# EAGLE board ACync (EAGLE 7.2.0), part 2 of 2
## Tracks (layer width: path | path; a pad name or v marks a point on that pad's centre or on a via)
16VAC
  Top 0.5: R46.1 13.88,51.88 13.88,55 D1.K+ 13.88,55.12 13.88,57.75 | 13.88,57.75 13.88,61 D2.A- | F1.2A 7.88,62.75 7.88,57.75 F1.2B 8.12,57.75 13.88,57.75
!ADC_CS  (via drill 0.51)
  Top 0.18: v267.88,41.88 267.88,40.88 267.38,40.38 v244.5,40.38 243,40.38 IC3.19 | v278.88,43.88 279.12,43.88 281,42 281,40.62 281.38,40.25 282.88,40.25 IC4.19 | v143.75,64 143.5,63.75 142.38,63.75 IC20.67 | v227.93,44.12 v195.64,44.12
  Bottom 0.18: v267.88,41.88 276.88,41.88 v278.88,43.88 | v195.64,44.12 163.38,44.12 156.64,50.86 156.64,59.64 155.64,60.64 147.36,60.64 144,64 v143.75,64 | v244.5,40.38 244.5,40.88 244.08,41.3 244.08,44.64 243,45.72 240.12,45.72 238.53,44.12 v227.93,44.12
!DAC_CS  (via drill 0.51)
  Top 0.18: v157.88,62.25 142.38,62.25 IC20.64 | v169.62,59.75 170.75,60.88 170.75,61.5 IC12.23
  Bottom 0.18: v169.62,59.75 160.38,59.75 v157.88,62.25
!DAC_LD  (via drill 0.51)
  Top 0.18: v155.62,65.5 152.88,62.75 142.38,62.75 IC20.65 | v165.25,65.5 169.5,69.75 169.5,70.38 IC12.7
  Bottom 0.18: v155.62,65.5 155.9,65.5 156.24,65.16 164.91,65.16 v165.25,65.5
!POT_STRT  (via drill 0.51)
  Top 0.18: v109.38,52.62 115,58.25 120.5,58.25 IC20.125 | v49,20.38 47.5,20.38 47.25,20.12 IC15.7
  Bottom 0.18: v109.38,52.62 101.2,52.62 101.2,52.6 97.2,48.6 97.2,41.76 95.76,40.32 92.07,40.32 71.12,19.38 50,19.38 v49,20.38
+1.2V  (via drill 0.51)  (1 unrouted)
  Top 0.25: v122.04,66.24 122.02,66.26 IC20.109 120.5,66.32 | IC20.102 126.11,66.85 v126.36,66.6 | IC20.116 121.44,62.76 v122.04,63.38 | IC20.124 121.24,58.76 121.68,58.59 v122.04,58.32 | IC20.138 121.42,51.76 v122.22,52.56 | IC20.5 125.11,47.69 v125.28,47.88 | IC20.1 123.11,47.51 v123.12,47.88 | IC20.29 137.11,47.83 v137.16,47.88 | IC20.45 140.96,52.76 v140.76,52.56 | IC20.78 138.11,67.09 v138.6,66.6 | IC20.84 135.11,66.71 v135,66.6 | C97.2 140.61,68.62 IC20.73 140.95,68.21 v141.12,68.04 | IC20.38 IC20.37 143.82,48.76 C86.2 | IC20.34 139.61,47.59 v139.32,47.88 | IC20.70 140.86,65.26 v140.76,65.16
  Top 0.4: 120.5,66.8 120.5,66.32
  Top 0.5: IC20.37 142.2,48.82 v142.2,48.96 | C50.2 101.12,62 101.12,65 C47.2 | C47.2 IC16.2 | C47.2 101.25,65.12 102.75,66.62 102.78,66.6 104.4,66.6 105.2,67.4 119.9,67.4 120.5,66.8
  Bottom 0.25: v122.04,66.24 C91.2 | v126.36,66.6 C90.2 | v122.04,63.38 C92.2 | v122.04,58.32 C94.2 | v122.22,52.56 C93.2 | v125.28,47.88 C83.2 | v123.12,47.88 C95.2 | v137.16,47.88 C85.2 | v140.76,52.56 C87.2 | v138.6,66.6 C89.2 | v135,66.6 C98.2 | v139.32,47.88 C96.2 | C88.2 140.72,65.2 v140.76,65.16
  Bottom 0.5: v122.04,58.32 120.96,59.4 120.96,63 121.32,63.36 122.02,63.36 v122.04,63.38 v122.04,66.24 122.04,66.96 122.76,67.68 125.62,67.68 126.36,66.94 v126.36,66.6 126.36,66.96 127.08,67.68 134.75,67.68 135.11,67.32 | C94.2 120.96,57.02 120.96,53.28 121.68,52.56 | 121.68,52.56 v122.22,52.56 | 121.68,52.56 120.96,51.84 120.96,48.96 122.04,47.88 v123.12,47.88 v125.28,47.88 126.36,46.8 136.75,46.8 137.11,47.16 137.11,47.83 v137.16,47.88 v139.32,47.88 141.12,47.88 v142.2,48.96 142.2,51.48 141.48,52.2 141.12,52.2 v140.76,52.56 | 135.11,67.32 135.47,67.68 137.86,67.68 138.6,66.94 v138.6,66.6 140.02,66.6 | 135.11,67.32 135.11,66.71 v135,66.6 | 140.02,66.6 140.76,65.86 v140.76,65.16 | 140.02,66.6 141.12,67.7 v141.12,68.04
+2.5V  (via drill 0.51, 0.71)  (1 unrouted)
  Top 0.25: 128.61,66.87 v128.88,66.6 | IC20.107 123.61,69.53 C78.2 | IC20.75 139.61,69.19 139.32,69.48 139.32,69.7 C81.2 | IC20.35 140.11,45.29 140.32,45.08 140.4,45 140.9,45 C80.2 | IC20.3 124.11,45.23 C84.2
  Top 0.5: R42.2A 135.62,33.25 136.38,33.25 R42.3A 136.38,33 136.38,32.62 136.75,32.25 137.62,32.25 138.88,33.5 138.88,33.75 140,34.88 C65.2 139.5,34.62 136.62,37.5 J15.4 136.62,37.75 137.75,38.88 137.75,41 138,41.25 | 138,41.25 140.25,43.5 140.25,45 140.32,45.08 | IC11.2 C39.2 101.12,54 101.12,51 C49.2 101,50.88 v101,50.45 | v123.5,70.62 123.5,69.62 C78.2 | v139.12,71 139.12,69.88 C81.2 | v124.38,43.88 124.38,45 C84.2 | v140,64.12 130.38,64.12 129,65.5 129,66.5 v128.88,66.6 | v135.12,44.12 138,41.25
  Bottom 0.25: v128.88,66.6 C82.2
  Bottom 0.5: v123.5,70.62 123.75,70.62 124.12,70.25 | 124.12,70.25 125.75,68.62 138,68.62 139.12,69.75 | v139.12,71 139.12,69.75 | v124.38,43.88 124.38,44.5 123,45.88 | 123,45.88 120.25,48.62 120.25,49.38 | 120.25,49.38 120.25,66.38 124.12,70.25 | v140,64.12 141,64.12 142.12,65.25 142.12,68.38 140.88,69.62 139.25,69.62 139.12,69.75 | v135.12,44.12 133.25,46 123.12,46 123,45.88 | 120.25,49.38 102.08,49.38 v101,50.45
+3.3V  (via drill 0.51, 0.71)
  Top 0.25: IC20.130 122,55.76 v122.04,55.8 | IC20.139 122,51.26 v122.04,51.3 | IC20.17 131.11,47.81 v131.04,47.88 | IC20.26 135.61,47.63 v135.36,47.88 | IC20.40 141.07,50.26 v140.76,49.95 | IC20.47 140.79,53.76 v140.76,53.73 | IC20.62 140.82,61.26 v140.76,61.2 | IC20.93 130.61,66.67 v130.68,66.6 | IC20.117 122.02,62.26 v122.04,62.28 | IC20.56 141.06,58.26 v140.76,57.96 | IC20.81 136.61,66.79 v136.8,66.6 | IC20.122 121.86,59.76 v122.04,59.94 | R61.1 112.81,49.55 113.04,49.32 113.04,48.44 IC18.7
  Top 0.5: C58.1 110.27,48.22 111.12,48.22 | 111.12,48.22 IC18.8 112.12,48.25 113.25,48.25 IC18.7 113.38,48 113.38,46.25 114,45.62 | IC4.18 280.37,39.67 280.08,39.96 280.08,42.12 279.27,42.92 IC4.2 275.02,42.92 C32.1 274.75,43.12 268.56,49.32 237.38,49.32 | C30.1 235.03,42.92 IC3.2 238.38,42.92 | 238.38,42.92 239.68,42.92 240.12,42.48 240.12,40.32 | 240.12,40.32 240.76,39.67 IC3.18 | C48.2 233,67 233,64.12 C38.2 IC10.2 235.62,63.88 236.62,62.88 236.75,62.88 237.38,62.25 237.38,49.32 | 238.38,42.92 238.38,44.62 237.38,45.62 237.38,49.32 | R17.CW 41.38,5.5 39.12,7.75 39.12,18 40.88,19.75 C41.1 41.11,20.06 IC15.2 43.38,20.12 43.88,20.12 44.74,20.98 44.74,22.42 49.82,27.5 56.74,27.5 57.6,26.64 57.6,24.48 58.32,23.76 84.24,23.76 86.4,25.92 97.42,25.92 102.75,31.25 104,31.25 111.88,39.12 | 114,45.62 114.5,45.12 114.5,44.25 IC18.3 | R55.3B 120.62,33.25 121.38,33.25 R55.2B | R55.2B 121.62,33.25 122.12,33.25 R55.1B 122.38,33.12 124,33.12 C59.2 124.12,33.25 126,33.25 | J15.6 134,37.62 133,36.62 C66.2 132.88,34.75 131.38,33.25 131.25,33.25 | 131.25,33.25 126,33.25 | 126,33.25 v126,34.25 | 111.12,48.22 111.12,39.88 111.88,39.12 | 111.88,39.12 118.75,32.25 120.25,32.25 121.12,33.12 R55.2B | 131.25,33.25 131.25,33.12 133.24,31.14 139.76,31.14 144.88,36.25 144.88,38.25 IC19.4 IC19.1 149.16,38.52 150.12,38.52 151,39.4 C67.1 153.45,40.05 156.35,42.95 C60.1 161.29,42.95 IC21.24 161.64,42.35 161.64,40.68 164.42,37.9 195.4,37.9 197.75,40.25 v212.88,40.25 | v122.12,49.62 122.12,48.75 120.75,47.38 120.75,46.62 119.88,45.75 114.12,45.75 114,45.62 | v239.38,40.25 239.88,40.25 240.12,40.32
  Bottom 0.25: v122.04,59.94 C68.2 | v122.04,55.8 C69.2 | v122.04,51.3 C70.2 | v131.04,47.88 C71.2 | v135.36,47.88 C72.2 | v140.76,49.95 C73.2 | v140.76,53.73 C74.2 | v140.76,61.2 C76.2 | v130.68,66.6 C79.2 | C63.2 v122.04,62.28 | C75.2 v140.76,57.96 | C77.2 v136.8,66.6
  Bottom 0.5: v122.04,59.94 122.04,60.84 | 122.04,60.84 v122.04,62.28 | 122.04,60.84 123.84,60.84 124.56,60.12 124.56,58.32 v122.04,55.8 124.56,53.28 124.56,51.12 | 122.4,50.4 123.84,50.4 124.56,51.12 | 124.56,51.12 126,51.12 129.24,47.88 v131.04,47.88 134.28,47.88 | v135.36,47.88 134.28,47.88 | 134.28,47.88 134.28,50.04 135.36,51.12 137.88,51.12 138.24,51.48 | v140.76,49.95 140.76,50.76 140.4,51.12 138.6,51.12 138.24,51.48 | 138.24,51.48 138.24,54 138.96,54.72 140.4,54.72 | 140.4,54.72 140.76,54.36 v140.76,53.73 | 140.4,54.72 140.76,55.08 v140.76,57.96 140.76,60.12 | v140.76,61.2 140.76,60.12 | C77.2 136.84,66.42 137.34,66.42 137.79,65.97 137.79,64.53 137.34,64.08 137.16,64.08 | 137.16,64.08 132.48,64.08 131.76,64.8 131.76,66.24 131.4,66.6 v130.68,66.6 | 122.4,50.4 122.04,50.76 v122.04,51.3 | v126,34.25 122.62,37.62 J16.4 | v122.12,49.62 122.25,49.75 122.25,50.25 122.4,50.4 | v212.88,40.25 v239.38,40.25 | 140.76,60.12 137.52,60.12 137.52,63.72 137.16,64.08
+5V  (via drill 0.71)
  Top 0.4: IC4.3 278.12,42.27 278.28,42.12 | IC3.3 238.16,42.27 238.32,42.12
  Top 0.5: C61.1 100.76,32.05 IC22.24 | IC24.8 189.95,46.19 C64.2 189.36,47.59 189.36,53.38 | C23.2 C33.1 274.98,39.02 IC4.8 278.06,39.02 278.28,39.24 278.28,40.12 | 278.28,42.12 278.28,40.12 | C31.1 234.97,39.02 IC3.8 238.1,39.02 238.32,39.24 238.32,42.12 | 28.05,28.88 28.05,28.29 IC23.8 | R39.1 21.62,33 23.3,31.32 26.64,31.32 26.95,31.01 C62.2 28.05,28.9 28.05,28.88 | 28.05,28.88 30.5,28.88 31.38,29.75 44.38,29.75 45,29.12 45,28.88 IC17.5 45,28.62 46.5,28.62 47,28.12 C100.2 47.12,28.25 57.07,28.25 58.32,27 58.32,24.84 58.68,24.48 83.88,24.48 86.04,26.64 96.84,26.64 100.44,30.24 100.44,31.94 100.5,32 IC22.24 | C29.2 99,57 IC11.3 96.4,58.68 95.4,58.68 | IC22.24 100.25,32.75 100.25,34.75 96.12,38.88 84.75,38.88 83.5,40.12 83.5,52.55 89.63,58.68 95.4,58.68 | C55.2 198,61 198,63 C40.2 | C55.2 198.12,61.5 201,61.5 IC5.3 201.12,61.25 206.38,56 235.12,56 | 189.36,53.38 178.88,53.38 175.38,56.88 173.25,56.88 172.25,57.88 C27.1 172.1,58.05 IC12.24 172.1,65.14 170.84,66.41 IC12.6 170.75,70.62 170.75,71.25 v169.62,72.38 | C19.2 235,37 235,38.88 C31.1 | C28.2 235,61 IC10.3 235.12,60.88 235.38,60.62 v235.38,58 235.12,57.75 235.12,56 | C31.1 234.88,39.25 234.88,41.38 234.12,42.12 234.12,44.75 235.12,45.75 235.12,56 | v278.38,40.12 278.28,40.12 | v122.75,77 110.12,77 101.25,68.12 C46.2 99,68 IC16.3 95.98,67.54 95.4,66.96 95.4,58.68 | C55.2 197.95,56.83 194.5,53.38 189.36,53.38
  Bottom 0.5: v122.75,77 123.25,77 124.75,78.5 163.5,78.5 v169.62,72.38 | v235.38,58 242.38,58 261.38,39 276,39 277.12,40.12 v278.38,40.12
+10V
  Top 0.18: IC13.1 181,71 R1.1 181,71.12 179,71.12 C34.2 179,71 178.5,70.5 177.25,70.5 IC12.1
+15V  (via drill 0.71)  (2 unrouted)
  Top 0.5: IC1.8 232.05,28.29 C1.2 232.25,30.12 233.25,31.12 238.75,31.12 242.25,34.62 C18.2 | IC14.8 252.05,28.29 C42.2 252.25,30.12 252.56,30.44 | IC2.8 272.03,29.98 C3.2 | IC9.8 292.05,28.29 291.87,28.47 C44.2 291.87,31.05 290.52,32.4 284.76,32.4 284.4,32.76 281.88,32.76 281.77,32.87 | IC4.15 282.17,37.73 281.88,37.44 281.88,35.17 C22.2 282,34.95 282,33.1 281.77,32.87 | IC3.15 242.21,37.73 241.92,37.44 | 241.92,37.44 241.92,35.13 C18.2 | C18.2 242.25,34.88 245.12,32 251,32 252.56,30.44 | C3.2 272.25,30.12 273.25,31.12 274.56,31.12 275.6,30.08 278.98,30.08 281.77,32.87 | 252.56,30.44 254.88,32.75 269.25,32.75 271.88,30.12 C3.2 | C56.2 74,55 72,55 C9.2 72.62,55.12 72.62,58 IC6.3 72.75,58.12 v83.28,58.12 | IC12.25 173.38,60.75 174,60.12 C35.2 174.12,58.12 183.38,58.12 183.5,58 185.38,58 195.62,68.25 | 197.88,66 195.62,68.25 | 195.62,68.25 189.88,74 v180,74 180.88,73.12 R1.2 181,72.88 | v239.62,37.5 241.75,37.5 241.92,37.44
  Bottom 0.5: v83.28,58.12 83.62,58.12 105.5,80 174,80 v180,74 180.12,73.88 180.12,67.5 210.12,37.5 v239.62,37.5
-10V
  Top 0.18: 181,61 IC8.2 | 181,61 179,61 | 181,61 R2.2 | 179,61 178.5,61.5 177.25,61.5 IC12.28 | 179,61 C36.2
-15V  (via drill 0.71)  (1 unrouted)
  Top 0.25: IC4.10 276.05,37.73 275.67,37.35 275.67,36.27 275.04,35.64 275.04,35.05 C25.1 | IC3.10 236.09,37.73 235.8,37.44 235.8,36 234.95,35.15 C21.1
  Top 0.5: IC1.4 227.95,24.44 C2.2 228.12,23.38 230.5,23.38 | 287.95,24.44 IC9.4 | 230.5,23.38 244.75,23.38 245.5,24.12 247.75,24.12 IC14.4 247.95,24.44 C43.2 248.12,23.5 253.25,23.5 253.8,24.05 253.8,24.48 254.16,24.84 266.4,24.84 266.78,24.46 IC2.4 267.95,24.44 C4.2 268.12,23.62 273.38,23.62 274,24.25 279.12,24.25 | 279.12,24.25 279.38,24.25 279.5,24.12 287.75,24.12 IC9.4 | 232.25,31.88 233.62,31.88 233.88,32.12 233.88,33.62 234.88,34.62 234.88,35 C21.1 | 232.25,31.88 230.5,30.12 230.5,23.38 | v278.38,37.12 277.75,37.75 277.12,37.75 IC4.10 | v279.12,24.5 279.12,24.25 | C57.1 66,49.12 68,49.12 C10.2 | C10.2 67.38,49 67.38,46 IC7.3 | R2.1 181,59.12 182.62,59.12 183.5,60 185.5,60 185.75,60.25 185.88,60.25 v186,60.12 186.35,60.48 186.84,60.48 190.08,63.72 190.08,64.08 187.16,67 176,67 173.38,69.62 IC12.4 173.25,70.62 173,70.88 173,74 C13.1 172.75,74.12 v171.38,75.5 | v74.25,49.88 69.12,49.88 68.25,49 C10.2 | v210.88,35.25 229.12,35.25 232.12,32.25 232.12,32 232.25,31.88 | C45.2 287.97,22.8 IC9.4
  Bottom 0.5: v74.25,49.88 76.73,49.88 106.11,79.25 167.62,79.25 v171.38,75.5 | v186,60.12 v210.88,35.25 | v278.38,37.12 280.44,35.06 280.44,26.28 279.12,24.96 v279.12,24.5
ADC1  (via drill 0.51)
  Top 0.18: v235.75,44.88 237,43.62 IC3.1 | v176.5,57.12 v193.88,57.12 | v149.62,64.75 142.38,64.75 IC20.69
  Bottom 0.18: v193.88,57.12 206.12,44.88 224.88,44.88 226.44,46.44 234.19,46.44 v235.75,44.88 | v176.5,57.12 168.88,64.75 v149.62,64.75
ADC2  (via drill 0.51)
  Top 0.18: v241.38,42.88 242.88,42.88 IC3.23 | v212.12,42.88 197.25,42.88 194.5,40.12 179.88,40.12 160.75,59.25 142.38,59.25 IC20.58
  Bottom 0.18: v241.38,42.88 234.75,42.88 234.36,42.48 212.52,42.48 v212.12,42.88
ADC3  (via drill 0.51)
  Top 0.18: v266,53.38 275.75,43.62 277,43.62 IC4.1 | v256.25,63.12 255.75,63.12 241.12,77.75 152.75,77.75 149,74 149,70.88 143.88,65.75 142.38,65.75 IC20.71
  Bottom 0.18: v256.25,63.12 v266,53.38
ADC4  (via drill 0.51)
  Top 0.18: IC4.23 282.88,43 281.75,43 266.62,58.12 259.12,58.12 239.88,77.38 152.97,77.38 149.4,73.8 149.4,70.15 v148.75,69.5 | IC20.72 143.66,66.26 146.52,69.12 146.52,69.45 v146.47,69.5
  Bottom 0.18: v146.47,69.5 v148.75,69.5
ADC_!START  (via drill 0.51)
  Top 0.18: 245.62,41.62 245.78,41.62 245.91,41.5 v264.15,41.5 | 245.62,41.62 IC3.21 | v277,44.62 279.5,44.62 282.5,41.62 IC4.21 | v152.5,63.5 152.25,63.25 142.38,63.25 IC20.66 | 245.62,41.62 v245.62,41.5 | v194,47.12 221.12,47.12 v222.12,46.12
  Bottom 0.18: v277,44.62 267.28,44.62 v264.15,41.5 | v222.12,46.12 222.12,46.45 224.28,48.6 243,48.6 245.52,46.08 245.52,41.6 v245.62,41.5 | v152.5,63.5 153,63 159.48,63 162,60.48 170.15,60.48 184.5,46.12 193,46.12 v194,47.12
ADC_SCLK  (via drill 0.51)
  Top 0.18: v267,41.12 266.62,40.75 245.25,40.75 244.88,41.12 244.12,41.12 244,41 243,41 IC3.20 242.88,41 242.38,41 v241.75,41.62 | v281.75,41 282.88,41 IC4.20 | v140.75,63.12 140.75,63.62 141.38,64.25 IC20.68 | v225.69,41.62 v198.5,41.62
  Bottom 0.18: 281.62,41.12 v281.75,41 279.91,42.84 278.64,42.84 277.2,41.4 268.92,41.4 268.64,41.12 v267,41.12 | v241.75,41.62 241.34,41.62 240.48,42.48 235.44,42.48 234.36,41.4 225.91,41.4 v225.69,41.62 | v198.5,41.62 197.06,41.62 195.12,43.56 163.31,43.56 156,50.88 156,59 155,60 147,60 144,63 140.88,63 v140.75,63.12
AGND  (via drill 0.51, 0.71)  (21 unrouted)
  Top 0.18: IC20.118 121.48,61.76 121.77,61.47 123.03,61.47 123.48,61.92 v123.48,62.28 | IC20.123 121.55,59.26 121.68,59.13 123.21,59.13 123.48,59.49 v123.48,59.94 | IC20.131 121.5,55.26 121.77,54.99 123.03,54.99 123.48,55.44 v123.48,55.8 | IC20.140 121.5,50.76 121.77,50.49 123.21,50.49 123.48,50.76 v123.48,51.3 | IC20.19 132.11,48.61 131.76,48.96 131.4,48.96 v131.04,49.32 | IC20.27 136.11,48.93 135.72,49.32 v135.36,49.32 | IC20.41 139.68,50.76 139.32,50.4 v139.32,50.04 140.61,48.75 IC20.36 140.93,46.41 C80.1 | IC20.48 141.31,54.26 141.03,54.54 139.86,54.54 139.32,54 v139.32,53.64 | IC20.57 139.76,58.76 139.32,58.32 v139.32,57.96 | IC20.63 141.28,61.76 141.03,62.01 139.77,62.01 139.32,61.56 v139.32,61.2 | IC20.79 137.61,65.61 137.16,65.16 v136.8,65.16 136.44,65.16 135.99,65.61 135.99,67.05 136.11,67.17 IC20.82 | IC20.95 129.61,65.87 130.32,65.16 v130.68,65.16 | v123.48,66.24 123.11,66.61 IC20.108 123.11,68.77 122.76,69.12 122.76,69.38 C78.1 | IC20.4 124.61,47.47 124.56,47.52 124.11,47.52 | 124.11,47.52 123.84,47.52 123.61,47.29 IC20.2 123.61,45.27 C84.1 | IC20.74 140.11,69.77 C81.1 140.4,69.62 C97.1 | v123.84,49.32 123.93,49.32 124.11,49.14 124.11,47.52 | 16COM.TP 6.12,34.2 | 2.52,34.2 16COM.TP | 16COM.TP 4.32,36 | 4.32,32.4 16COM.TP
  Bottom 0.18: C63.1 v123.48,62.28 123.26,62.5 C92.1 | v123.48,59.94 C68.1 C94.1 | C69.1 v123.48,55.8 | v123.48,51.3 C70.1 C93.1 | C71.1 v131.04,49.32 | C72.1 v135.36,49.32 135.58,49.1 C85.1 C96.1 | C73.1 v139.32,50.04 | C74.1 v139.32,53.64 139.54,53.42 C87.1 | C75.1 v139.32,57.96 | C76.1 v139.32,61.2 | C77.1 v136.8,65.16 | C79.1 v130.68,65.16 130.46,65.38 C82.1 C90.1 | C91.1 v123.48,66.24 | C95.1 123.62,49.1 v123.84,49.32 124.06,49.1 C83.1 | 139.32,48.96 v139.32,50.04 | 139.54,50.26 v139.32,50.04 | 137.02,65.38 v136.8,65.16 | 136.58,65.38 v136.8,65.16 | C89.1 138.78,65.2 138.92,65.2 | 138.92,65.2 C88.1 | 138.92,65.2 v138.96,65.16 | v135,65.16 C98.1
  other vias: 36,27 32.04,30.96 72.72,46.08 68.04,51.84 98.72,51.56 108.44,46.16 116,44 103.04,57.04 158.84,41.12 158.84,33.2 150.92,41.84 185.12,70.64 177.56,73.16 191.6,38.96 191.6,41.12 178.84,59.2 172,55.96 168.76,66.04 233,38.96 233,35 235.08,27.96 236.96,33.2 247.04,35 253.88,29.96 235.88,41.48 241.28,38.6 118.52,36.44 122.48,36.28 126.38,36.38 141.5,35.3 100.16,49.04 102.68,48.32 103.04,54.08 274.04,29.96 272.96,32.84 276.2,32.84 278.12,35.12 175.76,40.4 175.76,36.44 126.36,65.16 45.36,19.08 265.76,23.12 24.84,29.88 23.76,24.12
  pour Top (rank 2): 0,0 300,0 300,81 0,81
  pour Bottom (rank 2): 0,0 300,0 300,81 0,81
  pour Top (rank 2): 0,0 300,0 300,81 0,81
  pour Bottom (rank 2): 0,0 300,0 300,81 0,81
ASDO  (via drill 0.51)
  Top 0.18: IC20.6 125.62,46.38 125.62,43.88 123.38,41.62 116.25,41.62 115,40.38 J16.9 | v116.88,47 116.88,47.12 115.88,48.12 IC18.5
  Bottom 0.18: v116.88,47 116.88,42.25 115,40.38 J16.9
CONF_DONE  (via drill 0.51)
  Top 0.18: R55.2A 121.5,34.88 121.5,39.25 122.5,40.25 J16.3 | v123.62,74.38 124,74 128.62,74 131.12,71.5 131.12,68.25 IC20.92 | v115.12,59 114.62,59 107.62,52 v107.62,48.38 107.28,48.03 CNFDN.TP
  Bottom 0.18: v123.62,74.38 123.62,73.88 120.96,71.21 120.96,69.48 120.24,68.76 117.72,68.76 115.2,66.24 115.2,59.08 v115.12,59 | J16.3 122.5,40.38 122.5,42.5 118.44,46.56 118.44,48.24 118.08,48.6 107.85,48.6 v107.62,48.38
D0  (via drill 0.51)
  Top 0.18: v119.12,55.25 119.62,54.75 120.5,54.75 IC20.132 | v112.62,65.62 v111,64 | v164.62,74.62 168.25,71 168.25,70.5 IC12.8
  Bottom 0.18: v119.12,55.25 117.62,53.75 115.88,53.75 109.5,60.12 109.5,62.5 v111,64 | v164.62,74.62 162.62,76.62 148.25,76.62 147,77.88 124.88,77.88 v112.62,65.62
D1  (via drill 0.51)
  Top 0.18: v118.38,57.5 118.38,54.88 119,54.25 120.5,54.25 IC20.133 | v146.62,77.12 v146.56,75.62 | v165.75,72.25 167,71 167,70.5 IC12.9
  Bottom 0.18: v146.56,75.62 126,75.62 121.32,70.94 121.32,69.12 120.6,68.4 118.08,68.4 115.56,65.88 115.56,60.12 115.92,59.76 117.82,59.76 118.38,59.2 v118.38,57.5 | v146.62,77.12 147.12,77.12 148,76.25 161.75,76.25 v165.75,72.25
D2  (via drill 0.51)
  Top 0.18: v117.25,54.5 118,53.75 120.5,53.75 IC20.134 | v113.75,65.62 v110.25,62.12 | v161.25,75.5 165.75,71 165.75,70.5 IC12.10
  Bottom 0.18: v117.25,54.5 116.75,54.5 116.62,54.38 115.88,54.38 110.25,60 v110.25,62.12 | v161.25,75.5 148.12,75.5 147.25,76.38 123.89,76.38 113.75,66.23 v113.75,65.62
D3  (via drill 0.51)
  Top 0.18: v143.14,69.02 141.25,67.12 139.38,67.12 139.12,67.38 139.12,68.12 IC20.76 | v164.38,68.5 164.38,70.38 IC12.11
  Bottom 0.18: v143.14,69.02 143.88,69.75 143.88,69.88 144.25,70.25 157.38,70.25 161.38,66.25 162.12,66.25 v164.38,68.5
D4  (via drill 0.51)
  Top 0.18: v138.12,70.12 138.62,69.62 138.62,68.25 IC20.77 | v162.5,72.12 162.5,71.75 163.12,71.12 163.12,70.5 IC12.12
  Bottom 0.18: v138.12,70.12 138.12,71.12 138.25,71.25 138.25,71.38 139,72.12 v162.5,72.12
D5  (via drill 0.51)
  Top 0.18: v137.12,70.75 137.12,68.25 IC20.80 | v160,72.88 161.88,71 161.88,70.5 IC12.13
  Bottom 0.18: v137.12,70.75 137.88,71.5 137.88,71.62 138.75,72.5 159.62,72.5 v160,72.88
D6  (via drill 0.51)
  Top 0.18: v156.38,74.75 160.62,70.5 IC12.14 | IC20.83 135.62,68.25 135.62,71.38 135,72 133.94,72 v133.66,72.28
  Bottom 0.18: v156.38,74.75 153.5,74.75 152.75,74 135.38,74 v133.66,72.28
D7  (via drill 0.51)
  Top 0.18: v116.25,55.12 116.25,54.38 117.38,53.25 120.5,53.25 IC20.135 | v121.38,75.5 142.62,75.5 144.62,73.5 v144.62,69.5 | v147.5,66.62 156.34,66.62 160.68,62.3 IC12.15
  Bottom 0.18: v116.25,55.12 115.75,55.12 111.75,59.12 111.75,65.88 112.83,66.96 113.4,66.96 121.38,74.94 v121.38,75.5 | v147.5,66.62 v144.62,69.5
D8  (via drill 0.51)
  Top 0.18: v134.88,69.62 134.62,69.38 134.62,68.25 IC20.85 | v137.12,71.88 140,71.88 v140.5,71.38 | v152.62,71.38 161.88,62.12 161.88,61.62 IC12.16
  Bottom 0.18: v137.12,71.88 v134.88,69.62 | v152.62,71.38 v140.5,71.38
D9  (via drill 0.51)
  Top 0.18: v134.88,70.75 134.12,70 134.12,68.25 IC20.86 | v154.75,73.25 154.75,70.62 163.12,62.25 163.12,61.62 IC12.17
  Bottom 0.18: v134.88,70.75 137.38,73.25 v154.75,73.25
D10  (via drill 0.51)
  Top 0.18: v133.62,70.62 133.62,68.25 IC20.87 | v153.88,74 155.12,74 156,73.12 156,70.62 164.38,62.25 164.38,61.62 IC12.18
  Bottom 0.18: v133.62,70.62 136.25,73.25 136.75,73.25 137.12,73.62 153.5,73.62 v153.88,74
D11  (via drill 0.51)
  Top 0.18: v128.12,69.62 128.12,68.25 IC20.98 | v161.75,67 161.75,66.12 165.75,62.12 165.75,61.62 IC12.19 | v132.25,73.75 141.53,73.75 142.2,73.08 142.2,70.8 v142.38,70.62
  Bottom 0.18: v132.25,73.75 v128.12,69.62 | v142.38,70.62 158.12,70.62 v161.75,67
DAC_A0
  Top 0.18: IC20.59 142.38,59.75 168.38,59.75 169.5,60.88 169.5,61.5 IC12.22
DAC_A1
  Top 0.18: IC20.60 142.38,60.25 160.12,60.25 160.25,60.12 167.5,60.12 168.25,60.88 168.25,61.5 IC12.21
DATA0
  Top 0.18: IC20.13 129.12,46.38 129.12,44.5 126.12,41.5 126.12,39.5 125.88,39.25 124.38,39.25 123.5,40.12 123.5,40.75 123,41.25 118.38,41.25 117.5,40.38 J16.7 117.38,40.25 116.38,39.25 114.5,39.25 113.38,40.38 113.38,44.12 IC18.2
DCLK  (via drill 0.51)
  Top 0.18: IC20.12 128.62,46.38 128.62,44.62 125.12,41.12 125.12,40.38 J16.1 | v119.75,47 117.12,49.62 115.25,49.62 114.62,49 114.62,48.25 IC18.6
  Bottom 0.18: v119.75,47 119.75,46.5 125,41.25 125,40.38 J16.1
N$1
  Top 0.18: IC3.16 244.38,38.38 245,39 C20.2
N$2
  Top 0.18: IC3.9 237.5,38.38 239.62,36.25 239.62,33.62 239,33 C11.2
N$3  (via drill 0.51)
  Top 0.18: 238.31,36.31 238.88,35.75 238.88,35 C14.2 | 238.31,36.31 237.62,37 237.12,37 IC3.11 | v228,32 R5.2 | v238.25,36.25 238.31,36.31
  Bottom 0.18: v228,32 234,32 v238.25,36.25
N$4  (via drill 0.51)
  Top 0.18: 245,37 243,37 IC3.14 | v241.88,31.88 236,26 R6.2 | 245,37 v246,36 | 245,37 C15.2
  Bottom 0.18: v246,36 v241.88,31.88
N$5
  Top 0.18: IC3.13 243,36.38 244,36.38 245,35.38 245,35 R14.2
N$6
  Top 0.18: IC3.12 236.94,36.42 236.16,35.64 236.16,34.21 R7.2
N$7
  Top 0.18: IC3.22 246.28,42.27 BUSY2.TP
N$8
  Top 0.18: R5.1 228,28.38 IC1.1 228,28.25 228,27 IC1.2
N$9  (via drill 0.51)
  Top 0.18: C51.2 244.12,29 244.12,27 R20.2 244,27 v244,25.5 | R12.2 235,13 234,12 230.09,12 J1.LWR-CTR
  Bottom 0.18: v244,25.5 244,24.38 231.62,12 230,12 J1.LWR-CTR
N$10
  Top 0.18: R6.1 232.38,26 232.12,25.75 IC1.6 232.12,25.88 232.12,27 IC1.7
N$11
  Top 0.18: R3.2 230,21 228.5,21 226.75,22.75 226.75,23.75 226.5,24 226.5,24.88 227.25,25.62 227.88,25.62 IC1.3
N$12  (via drill 0.51)
  Top 0.18: v237.12,22.38 238.5,21 250,21 R4.2 | v235.12,24.38 232.12,24.38 IC1.5
  Bottom 0.18: v235.12,24.38 v237.12,22.38
N$13  (1 unrouted)
  Top 0.18: J2.UPR-CTR R4.1
N$14  (1 unrouted)
  Top 0.18: J1.UPR-CTR R3.1
N$15  (via drill 0.51)
  Top 0.18: 256,26 256,28 C52.2 | v257,26 256,26 | 256,26 R21.2 | R13.2 255,13 254,12 250.09,12 J2.LWR-CTR
  Bottom 0.18: v257,26 257,20.5 251.12,14.62 251.12,13.12 250,12 J2.LWR-CTR
N$16
  Top 0.18: R21.1 252.38,26 252.12,25.75 IC14.6
N$17
  Top 0.18: R23.1 292.38,26 292.12,25.75 IC9.6
N$18  (via drill 0.51)
  Top 0.18: v237.62,20.75 R12.1 | C51.1 245.88,29 v245,28.12 245.38,28.38 247.88,28.38 IC14.1
  Bottom 0.18: v245,28.12 243.12,28.12 241,26 241,24.12 v237.62,20.75
N$19  (via drill 0.51)
  Top 0.18: v255,23.25 R13.1 | v255,27.12 254.12,28 C52.1 254,28 253,27 IC14.7
  Bottom 0.18: v255,27.12 v255,23.25
N$20
  Top 0.18: IC9.2 R22.1
N$21
  Top 0.18: IC14.2 R20.1
N$22  (via drill 0.51)
  Top 0.18: C53.2 284.12,29 284.12,27 R22.2 284,27 v284,25.5 | R18.2 275,13 274,12 270.09,12 J3.LWR-CTR
  Bottom 0.18: v284,25.5 284,20.38 275.62,12 270,12 J3.LWR-CTR
N$23
  Top 0.18: C54.2 296,28 296,26 R23.2 295.88,26 295.88,20.14 295,19.27 R19.2 295,13.38 293.62,12 290,12 J4.LWR-CTR
N$24  (via drill 0.51)
  Top 0.18: v276.19,20.75 R18.1 | IC9.1 285.84,28.27 | 285.84,28.27 285.14,28.27 v285,28.12 | C53.1 285.95,28.38 285.84,28.27
  Bottom 0.18: v285,28.12 284.95,28.08 283.32,28.08 282.24,27 282.24,22.32 280.67,20.75 v276.19,20.75
N$25
  Top 0.18: R19.1 295,27.12 294.12,28 C54.1 293.05,27 IC9.7
N$26  (via drill 0.51)  (2 unrouted)
  Top 0.18: v249.75,24.5 252,24.5 IC14.5 | v176.88,68 176.88,69 176,69.88 176,70.38
  Bottom 0.18: v249.75,24.5 249.75,27.25 247,30 213,30 196.56,46.44 196.56,47.36 192.44,51.48 191.52,51.48 176.88,66.12 v176.88,68
N$27  (via drill 0.51)  (2 unrouted)
  Top 0.18: v236.62,24.75 244.38,24.75 245.25,25.62 247.88,25.62 IC14.3 | v175.88,68.62 174.75,69.75 174.75,70.38
  Bottom 0.18: v236.62,24.75 237,25.12 237,26 236.12,26.88 215.38,26.88 215.38,26.91 196.2,46.08 196.2,47.16 192.24,51.12 191.16,51.12 175.88,66.41 v175.88,68.62
N$28  (via drill 0.51)  (2 unrouted)
  Top 0.18: v278.12,27 280.38,24.75 284.38,24.75 285.25,25.62 287.88,25.62 IC9.3 | v187.08,63 176.88,63 176,62.12 176,61.62
  Bottom 0.18: v278.12,27 265.12,27 251,41.12 251,44 243,52 233,52 222,63 v187.08,63
N$29  (via drill 0.51)  (2 unrouted)
  Top 0.18: v290.83,24.32 291.38,24.5 292,24.5 IC9.5 | v185.84,64.95 177.46,64.95 174.75,62.25 174.75,61.62
  Bottom 0.18: v185.84,64.95 273.92,64.95 290.83,48.05 v290.83,24.32
N$30
  Top 0.18: IC4.16 284.75,38.38 285,38.62 C24.2
N$31
  Top 0.18: IC4.9 278.38,38.38 279.25,37.5 279.25,34.25 278,33 C12.2
N$32  (via drill 0.51)
  Top 0.18: IC4.11 276.48,37.08 276.12,36.72 276.12,35.15 C16.2 275.88,34.88 275.88,34.5 275.38,34 v271.88,34 | v268.88,31 268,31.88 R10.2
  Bottom 0.18: v271.88,34 v268.88,31
N$33  (via drill 0.51)
  Top 0.18: 285,37 283,37 IC4.14 | 285,37 v286,36 | R11.2 276,26 278,28 280,28 v283,31 | 285,37 C17.2
  Bottom 0.18: v286,36 283,33 v283,31
N$34
  Top 0.18: IC4.13 283,36.38 284,36.38 285,35.38 285,35 R16.2
N$35
  Top 0.18: IC4.12 277.07,32.27 276.48,31.68 275.76,31.68 275.04,32.4 275.04,32.91 R15.2
N$36
  Top 0.18: IC4.22 286.27,42.27 BUSY3.TP
N$37
  Top 0.18: R10.1 268,28.38 IC2.1 268,28.25 268,27 IC2.2
N$38
  Top 0.18: R11.1 272.38,26 272.12,25.75 IC2.6 272.12,25.88 272.12,27 IC2.7
N$39  (via drill 0.51)
  Top 0.18: v270,21.18 R8.2 | IC2.3 268,25.62 269.57,25.62 v269.64,25.56
  Bottom 0.18: v269.64,25.56 270,25.2 v270,21.18
N$40  (via drill 0.51)
  Top 0.18: v280,22.25 281.25,21 290,21 R9.2 | v277,25.25 276.62,25.25 276.25,24.88 272.5,24.88 272.12,24.5 IC2.5
  Bottom 0.18: v280,22.25 277.63,22.25 277.2,22.68 277.2,25.05 v277,25.25
N$41  (1 unrouted)
  Top 0.18: J4.UPR-CTR R9.1
N$42  (1 unrouted)
  Top 0.18: J3.UPR-CTR R8.1
N$43  (via drill 0.51)
  Top 0.18: v138.88,43.5 138.12,44.25 138.12,46.38 IC20.31 | IC21.23 163,42.5 163,43.48 160.09,46.4 154.77,46.4 v151.88,43.5
  Bottom 0.18: v151.88,43.5 v138.88,43.5
N$44
  Top 0.18: IC20.39 142.38,49.75 158.34,49.75 164.25,43.84 164.25,42.5 IC21.22
N$45
  Top 0.18: IC20.42 142.38,51.25 158.46,51.25 165.5,44.2 165.5,42.5 IC21.21
N$46
  Top 0.18: IC20.43 142.38,51.75 158.84,51.75 166.75,43.84 166.75,42.5 IC21.20
N$47
  Top 0.18: J6.LWR-CTR 14.07,11.91 15.12,12.96 15.12,19.13 R51.2
N$48
  Top 0.18: R51.1 15,34.38 16.38,35.75 57.75,35.75 58.32,35.18 58.32,33.48 63.67,28.12 80.12,28.12 87.12,35.12 98.12,35.12 99,34.25 99,32.62 IC22.23
N$49
  Top 0.18: J14.LWR-CTR 63.91,11.91 65,13 R29.2
N$50
  Top 0.18: J13.LWR-CTR 83.91,11.91 85,13 R28.2
N$51
  Top 0.18: J12.LWR-CTR 103.91,11.91 105,13 R27.2
N$52
  Top 0.18: J11.LWR-CTR 123.91,11.91 125,13 R26.2
N$53
  Top 0.18: J10.LWR-CTR 143.91,11.91 145,13 R25.2
N$54
  Top 0.18: J9.LWR-CTR 163.91,11.91 165,13 R41.2
N$55
  Top 0.18: J8.LWR-CTR 183.91,11.91 185,13 R53.2
N$56  (1 unrouted)
  Top 0.18: J14.UPR-CTR R44.1
N$57
  Top 0.18: R31.2 200,21 185.88,21 185.47,21.41 183.11,21.41 172,32.52 172,33.5 IC21.9
N$58
  Top 0.18: J7.LWR-CTR 203.91,11.91 205,13 R52.2
N$59  (via drill 0.51)
  Top 0.18: R52.1 201.25,20.75 200.5,20 197,20 186,9 157.88,9 v148.88,18 | IC22.22 97.75,30.75 v97,30
  Bottom 0.18: v97,30 96.84,29.84 96.84,25.56 99,23.4 106.92,23.4 110.32,20 146.88,20 v148.88,18
N$60  (via drill 0.51)
  Top 0.18: R53.1 182.88,20.75 171.25,32.38 171.25,34.88 171.12,35 149.25,35 142.75,28.5 128,28.5 125.88,30.62 v109.75,30.62 | v97.75,34.38 96.5,33.12 96.5,32.62 IC22.21
  Bottom 0.18: v109.75,30.62 101.5,30.62 v97.75,34.38
N$61  (via drill 0.51)
  Top 0.18: IC22.20 95.2,31.67 v96.12,30.75 | R41.1 164.75,21 v164.75,21.75
  Bottom 0.18: v96.12,30.75 97.38,30.75 97.92,30.2 97.92,25.56 99.36,24.12 107.28,24.12 110.65,20.75 163.75,20.75 v164.75,21.75
N$62  (via drill 0.51)
  Top 0.18: v140.75,16.5 R25.1 | IC22.19 94,32.5 94,31.25 v94.5,30.75
  Bottom 0.18: v140.75,16.5 140.33,16.92 104.5,16.92 104.14,17.28 104.14,21.14 103.68,21.6 102.96,21.6 102.6,21.24 94.32,21.24 93.6,21.96 93.6,29.85 v94.5,30.75
N$63  (via drill 0.51)
  Top 0.18: v117.62,28.12 R26.1 | v96,34.25 92.93,34.25 92.67,33.98 IC22.18
  Bottom 0.18: v96,34.25 101.81,28.44 117,28.44 117.31,28.12 v117.62,28.12
N$64  (via drill 0.51)
  Top 0.18: v103.38,20.75 R27.1 | IC22.17 91.39,31 91.8,30.6 93.22,30.6 v93.38,30.75
  Bottom 0.18: v103.38,20.75 94.09,20.75 93.24,21.6 93.24,30.61 v93.38,30.75
N$65  (via drill 0.51)
  Top 0.18: v87.75,23.5 R28.1 | IC22.16 90.12,31.45 88.2,29.52 87.86,29.52 v87.75,29.62
  Bottom 0.18: v87.75,29.62 v87.75,23.5
N$66  (via drill 0.51)
  Top 0.18: v77.62,20.75 R29.1 | IC22.15 88.86,31.25 88.2,30.6 87.78,30.6 v87.62,30.75
  Bottom 0.18: v87.62,30.75 v77.62,20.75
N$67  (1 unrouted)
  Top 0.18: J13.UPR-CTR R56.1
N$68  (via drill 0.51)
  Top 0.18: v127.12,72.38 127.12,68.25 IC20.100 | v126.25,74.75 124.38,74.75 124,75.12 122.12,75.12 121.52,74.52 120.96,74.52 119.88,75.6 116.64,75.6 115.42,74.38 v115.25,74.38 | v90.12,43.25 88.88,42 88.88,41.5 IC22.10
  Bottom 0.18: v127.12,72.38 127.12,73.88 v126.25,74.75 | v115.25,74.38 90.12,49.25 v90.12,43.25
N$69  (via drill 0.51)
  Top 0.18: v125.88,69.88 125.62,69.62 125.62,68.25 IC20.103 | v116.45,65.62 114.88,65.62 114.05,64.8 113.56,64.8 111,62.23 111,61.75 104.5,55.25 97.38,55.25 96.45,54.33 96.45,48.33 90.12,42 IC22.9
  Bottom 0.18: v125.88,69.88 125.5,69.88 123.88,71.5 123.12,71.5 121.68,70.06 121.68,68.76 120.96,68.04 118.44,68.04 116.45,66.05 v116.45,65.62
N$70  (via drill 0.51)
  Top 0.18: v115.25,71.62 117.62,74 118.38,74 119.75,72.62 124.27,72.62 125.12,71.77 125.12,68.25 IC20.104 | v92.62,43.25 91.5,42.12 91.5,41.5 IC22.8
  Bottom 0.18: v115.25,71.62 92.62,49 v92.62,43.25
N$71  (via drill 0.51)
  Top 0.18: v93.88,43.25 92.75,42.12 92.75,41.5 IC22.7 | IC20.105 124.62,68.25 124.62,69.88 124.75,70 124.75,71.52 124.27,72 119.16,72 118,73.16 v118,73.25
  Bottom 0.18: v118,73.25 115.27,70.52 114.77,70.52 93.88,49.62 v93.88,43.25
N$72  (via drill 0.51)
  Top 0.18: v119.88,69.62 121.75,71.5 123.88,71.5 124.38,71 124.38,70.25 124.12,70 124.12,68.25 IC20.106 | IC22.6 94,41.5 94,42 99.88,47.88 100.75,47.88 101.88,49 101.88,51.38 112.5,62 112.61,62 v112.86,62.25
  Bottom 0.18: v119.88,69.62 119.88,69.47 119.52,69.12 117.36,69.12 114.84,66.6 114.84,63 114.12,62.28 112.89,62.28 v112.86,62.25
N$73
  Top 0.18: IC20.110 118.68,65.76 104.76,51.84 104.76,46.8 104.04,46.08 98.64,46.08 95.4,42.84 95.4,41.61 IC22.5
N$74
  Top 0.18: IC20.111 120.5,65.25 119,65.25 105.12,51.37 105.12,46.44 104.4,45.72 99.47,45.72 96.5,42.75 96.5,41.5 IC22.4
N$75
  Top 0.18: IC20.44 142.38,52.25 159.24,52.25 168,43.48 168,42.5 IC21.19
N$76
  Top 0.18: IC20.112 120.5,64.75 119.12,64.75 105.48,51.1 105.48,46.08 104.76,45.36 99.73,45.36 97.75,43.38 97.75,41.5 IC22.3
N$77
  Top 0.18: IC20.46 142.38,53.25 159.12,53.25 169.38,43 169.38,42.5 IC21.18
N$78
  Top 0.18: IC20.113 120.5,64.25 119.25,64.25 105.84,50.84 105.84,45.72 105.12,45 100,45 99.12,44.12 99.12,41.5 IC22.2
N$79
  Top 0.18: IC20.54 142.38,57.25 145.07,57.25 147.5,54.82 159.18,54.82 170.62,43.38 170.62,42.5 IC21.17
N$80
  Top 0.18: IC20.55 142.38,57.75 145.29,57.75 147.86,55.18 159.82,55.18 171.88,43.12 171.88,42.5 IC21.16
N$81
  Top 0.18: R39.2 19.12,33 19.12,31.75 20.88,30 R40.2 | IC23.6 28,25.75 27.38,25.75 25.38,27.75 25.38,28.62 25,29 22,29 21,30 R40.2 | 20.88,30.12 R40.2
N$82
  Top 0.18: R40.1 19.12,30 19.12,28.75 20.88,27 R24.2 IC23.2
N$83  (via drill 0.51)
  Top 0.18: v115.62,26 109.62,20 64.62,20 63.75,20.88 60,20.88 R44.2 | v155.88,26 163,33.12 163,33.5 IC21.2
  Bottom 0.18: v155.88,26 v115.62,26
N$84
  Top 0.18: R56.2 80,21 84.12,21 87.5,24.38 88.22,24.38 90.47,22.12 109.88,22.12 117,29.25 118.62,29.25 124.12,23.75 155,23.75 164.25,33 164.25,33.5 IC21.3
N$85
  Top 0.18: R57.2 100,21 102.5,21 103.25,21.75 110.12,21.75 117.25,28.88 118.23,28.88 123.73,23.38 156,23.38 165.5,32.88 165.5,33.5 IC21.4
N$86
  Top 0.18: R58.2 120,20.88 123.75,20.88 124.5,20.12 125.75,20.12 128.25,22.62 156.5,22.62 166.75,32.88 166.75,33.5 IC21.5
N$87
  Top 0.18: R59.2 140,21 140.12,21 141.38,22.25 157.38,22.25 168,32.88 168,33.5 IC21.6
N$88
  Top 0.18: R60.2 160,21 161.38,21 169.38,29 169.38,33.5 IC21.7
N$89
  Top 0.18: R30.2 180,23 170.75,32.25 170.75,33.5 IC21.8
N$90
  Top 0.18: 28.12,23.75 28.12,24.38 IC23.5 | 28.12,23.75 28.12,21.5 29.5,20.12 30.5,20.12 31.25,20.88 33,20.88 R38.2 | 28.12,23.75 26.25,25.62 24,25.62 IC23.3
N$91
  Top 0.18: R38.1 33,19.12 35,19.12 R37.2 34.92,18.97 34.92,13.32 33.51,11.91 J5.LWR-CTR
N$92  (via drill 0.51)
  Top 0.18: v28.12,31.38 28.12,33 R35.2 | v31.25,28.25 31.25,27.62 31.88,27 R33.2 | v143.75,55.25 143.25,55.75 142.38,55.75 IC20.51 | v101.88,27.38 100.25,27.38 97.66,24.78 87.06,24.78 84.96,22.68 56.45,22.68 v53.62,25.5
  Bottom 0.18: v28.12,31.38 v31.25,28.25 34,25.5 v53.62,25.5 | v143.75,55.25 146,55.25 155.38,45.88 155.38,38 144.75,27.38 v101.88,27.38
N$93  (via drill 0.51)
  Top 0.18: v25.92,33 R34.2 | v33,28 34,27 R36.2 | v146.12,54 143.88,56.25 142.38,56.25 IC20.52 | v102.12,29.25 101.5,29.25 97.42,25.17 86.73,25.17 84.6,23.04 57.6,23.04 56.52,24.12 56.52,26.23 v56.5,26.25
  Bottom 0.18: v25.92,33 28,33 v33,28 34.85,26.15 37.45,26.15 37.55,26.25 v56.5,26.25 | v102.12,29.25 146,29.25 155,38.25 155,45.12 v146.12,54
N$94  (via drill 0.51)
  Top 0.18: v57.38,35 44,35 R49.1 | v119,44.12 122.38,47.5 122.38,48.25 123,48.88 123,49.62 126.88,53.5 138.12,53.5 139.88,55.25 IC20.50 | v94.33,37.22 79.97,37.22 v79.25,36.5
  Bottom 0.18: v57.38,35 77.75,35 v79.25,36.5 | v94.33,37.22 112.97,37.22 115,39.25 115.01,39.24 115.56,39.24 115.92,39.6 115.92,40.68 119,43.76 v119,44.12
N$95  (via drill 0.51)
  Top 0.18: v143.75,54.12 143.12,54.75 142.38,54.75 IC20.49 | R50.1 42,34.88 42.27,34.88 43.03,34.11 57.12,34.11 63.48,27.75 82.38,27.75 v84.38,29.75
  Bottom 0.18: v84.38,29.75 84.88,29.75 90.62,35.5 99.5,35.5 102.6,32.4 144.36,32.4 145.08,33.12 149.04,33.12 154.44,38.52 154.44,45 146.52,52.92 144.96,52.92 v143.75,54.12
N$96
  Top 0.18: 43.12,31.88 43.12,32.12 44,33 R49.2 | 43.12,31.88 43.12,31.38 IC17.3 | 43.12,31.88 42,33 R50.2
N$97  (1 unrouted)
  Top 0.18: J12.UPR-CTR R57.1
N$98  (1 unrouted)
  Top 0.18: J6.UPR-CTR R45.1
N$99  (via drill 0.51)
  Top 0.18: R54.1 30.5,20.75 34.75,25 39.38,25 43,28.62 IC17.4 43.12,28.75 v44,28.75 | IC17.1 45,31.25 45.33,31.25 v45.38,31.2
  Bottom 0.18: v44,28.75 44,29.83 v45.38,31.2
N$100  (via drill 0.51)
  Top 0.18: v24.08,33 R34.1 | v24.08,28.25 24,28.38 IC23.1
  Bottom 0.18: v24.08,33 23.4,32.32 23.4,29.16 24.08,28.48 v24.08,28.25
N$101
  Top 0.18: IC23.7 R33.1
N$102
  Top 0.18: 60HZ.TP 184.97,47.67 IC24.1 184.88,45.25 182,45.25 | 182,45.25 182,46 R43.1 | 182,45.25 182,44 R32.2
N$103
  Top 0.18: R48.2 191.25,43 189.75,41.5 189.12,41.5 IC24.5 189,41.5 186.88,41.5 185.75,42.62 185,42.62 IC24.3 184.88,42.75 181.75,42.75 180.5,44 R32.1
N$104  (via drill 0.51)
  Top 0.18: R43.2 180.12,46 180.12,48 R47.2 180,48 v177.75,50.25 | IC20.53 142.38,56.75 144.85,56.75 147.6,54 v158.88,54
  Bottom 0.18: v158.88,54 174,54 v177.75,50.25
N$105  (1 unrouted)
  Top 0.18: J11.UPR-CTR R58.1
N$106  (via drill 0.51)
  Top 0.18: 194,43 D3.3 | v148.5,77.5 147.12,78.88 23.8,78.88 16.2,71.28 16.2,51.12 15.05,49.97 R46.2 | 193.88,45 C99.2 | 194,43 194,45 C99.2 | 194,43 R48.1 | v191.16,48.88 192.32,47.71 192.32,46.72 193.95,45.09 C99.2
  Bottom 0.18: v148.5,77.5 163.25,77.5 167.76,72.99 167.76,72 190.88,48.88 v191.16,48.88
N$107  (via drill 0.51)
  Top 0.18: v137.38,45 134.75,45 134.12,45.62 134.12,46.38 IC20.23 | v143.25,44.25 144.25,44.25 144.88,43.62 IC19.3
  Bottom 0.18: v137.38,45 138,45 138.75,44.25 v143.25,44.25
N$108
  Top 0.5: 16VAC.TP 4.32,38.95 F1.1A 7.88,42.62 7.88,47.5 F1.1B
N$109
  Top 0.18: J5.UPR-CTR R54.2
N$110
  Top 0.18: IC15.8 49.33,21.33 BUSY1.TP
N$111
  Top 0.5: D1.A- 23.75,55 C8.NEG 32.12,46.62 41.21,46.62 45.8,42.03 70,42.03 | C6.2 IC7.2 70,42.03 | IC7.TAB 70,42.03
N$112
  Top 0.5: C5.2 68,57.5 67.5,58 IC6.1 67.25,58.12 52.12,58.12 C7.POS 46,64.25 23.62,64.25 20.38,61 D2.K+
N$113
  Top 0.18: IC15.1 43.12,21.25 43,21.12 39,21.12 C26.2 39,18.62 38.5,18.12 38.5,5.25 40.5,3.25 42.38,3.25 46.5,7.38 46.5,8 R17.W
N$114  (via drill 0.51)
  Top 0.18: v139.12,45 139.12,46.38 IC20.33 | IC21.15 173.12,42.5 173.12,43.12 160.71,55.54 148.68,55.54 148.44,55.78 v148.44,57.5
  Bottom 0.18: v139.12,45 139.38,45 143,48.62 143,51.76 141.58,53.18 141.58,57.24 141.94,57.6 148.34,57.6 v148.44,57.5
N$115  (1 unrouted)
  Top 0.18: J10.UPR-CTR 139,15.45 139,18 140,19 R59.1
N$116  (1 unrouted)
  Top 0.18: J9.UPR-CTR R60.1
N$117  (1 unrouted)
  Top 0.18: J8.UPR-CTR R30.1
N$118  (1 unrouted)
  Top 0.18: J7.UPR-CTR R31.1
N$119
  Top 0.18: R61.2 LED1.1
N$120
  Top 0.18: IC20.144 118.64,48.76 117.72,49.68 117.72,50.63 LED1.2
N$121  (2 unrouted)
N$122  (via drill 0.51)
  Top 0.18: v10.88,20.88 10,20.88 R45.2 | v145.12,32 145.62,32 149,35.38 172,35.38 173.12,34.25 173.12,33.62 IC21.10
  Bottom 0.18: v10.88,20.88 37.62,20.88 42.62,15.88 71.62,15.88 90.88,35.12 98.62,35.12 101.75,32 v145.12,32
N$123  (1 unrouted)
N$124  (1 unrouted)
N$125  (1 unrouted)
N$126  (1 unrouted)
NCE  (via drill 0.51)
  Top 0.18: R55.4A 119.88,34.88 119.88,37.5 120,37.62 J16.6 | v133.12,44.62 133.12,46.38 IC20.21
  Bottom 0.18: v133.12,44.62 131.5,44.62 125.62,38.75 121,38.75 120,37.75 J16.6
NCONFIG
  Top 0.18: J16.5 120,40.25 121,39.25 121,37.38 120.62,37 120.62,34.88 R55.3A 120.62,34.75 120.62,34.38 121,34 124.5,34 125.78,35.28 127.08,35.28 127.69,35.88 127.69,40.44 129.62,42.38 129.62,46.38 IC20.14
NCSO  (via drill 0.51)
  Top 0.18: v126.62,44.88 126.62,46.38 IC20.8 | IC18.1 112,44.12 112,41.12 114.38,38.75 116.38,38.75 117.38,37.75 J16.8
  Bottom 0.18: v126.62,44.88 124.75,43 124,43 120.5,46.5 120.5,47.38 120.12,47.75 119.38,47.75 119,47.38 119,46.62 123.5,42.12 123.5,39.88 122.75,39.12 118.88,39.12 117.5,37.75 J16.8
NSTATUS  (via drill 0.51)
  Top 0.18: v127.75,42 126.75,41 126.75,38 125.5,36.75 124.38,36.75 122.5,34.88 122.25,34.88 R55.1A | v127.75,45 127.12,45.62 127.12,46.38 IC20.9
  Bottom 0.18: v127.75,45 v127.75,42
POT_CLK  (via drill 0.51)
  Top 0.18: v117.5,59 118.75,60.25 120.5,60.25 IC20.121 | v113.25,53.38 v117.25,57.38 | v88.62,43.25 v94.62,49.25 | v67,21.62 53.25,21.62 48.5,16.88 43.88,16.88 43.25,17.5 IC15.4
  Bottom 0.18: v117.5,59 117.5,57.62 v117.25,57.38 | v94.62,49.25 101.17,55.8 110.52,55.8 112.94,53.38 v113.25,53.38 | v67,21.62 v88.62,43.25
POT_DAT  (via drill 0.51)
  Top 0.18: v119.12,56.62 119.75,57.25 120.5,57.25 IC20.127 | v109.38,50.62 v115.38,56.62 | v99.88,43.75 100.8,44.64 105.48,44.64 106.56,45.72 106.56,50.44 v106.75,50.62 | v49,18.62 48,17.62 47.25,17.62 IC15.5
  Bottom 0.18: v115.38,56.62 v119.12,56.62 | v106.75,50.62 v109.38,50.62 | v99.88,43.75 95.88,39.75 92.12,39.75 71.36,18.98 49.36,18.98 v49,18.62
TCK  (via drill 0.51)
  Top 0.18: v130.88,42.75 130.62,43 130.62,46.38 IC20.16 | v138.25,34.5 137.2,33.45 R42.4A
  Bottom 0.18: v138.25,34.5 138.25,35.5 140.88,38.12 140.88,39.25 139.88,40.25 139.12,40.25 J15.1 139,40.38 136.62,42.75 v130.88,42.75
TDI  (via drill 0.51)
  Top 0.18: v133.88,34 135.25,34 135.5,34.25 135.5,34.75 R42.2B | IC20.15 130.12,46.38 130.12,41.5 129,40.38 J15.9
  Bottom 0.18: v133.88,34 131.12,36.75 131,36.75 129.88,37.88 129.88,39.38 129,40.25 J15.9
TDO
  Top 0.18: IC20.20 132.62,46.38 132.62,45.25 132.38,45 132.38,44.25 136.25,40.38 136.5,40.38 J15.3
TMS
  Top 0.18: R42.3B 136.38,34.88 136.38,35.25 135,36.62 135,39.25 134,40.25 J15.5 134,40.38 131.62,42.75 131.62,46.38 IC20.18

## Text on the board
tNames: ACync - AC Line Sync / University of Toronto / J. Thywissen Labs / Rev: A | AS | JTAG
Graphics: Check ref des origin, set to top centre.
